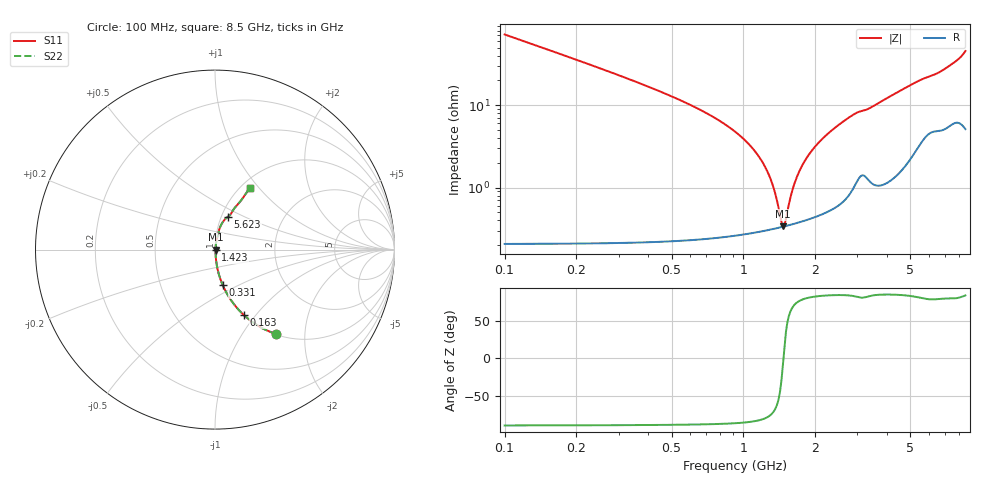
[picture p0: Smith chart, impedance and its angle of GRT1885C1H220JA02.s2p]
!Murata Part Number: GRT1885C1H220JA02
!These Parameters are Measured in Series Mode Connection
!Data Generated on Jun 19, 2026
!  o--ll--o
!Port1  Port2
!  o------o
!Operation Temp=25[degC], DC Bias Voltage=0[V]
!Freq. Start=100[MHz] Stop=9[GHz] 401[Steps]
# Hz S RI R 50
!Freq.(Hz) S11(Real) S11(Imag) S21(Real) S21(Imag) S12(Real) S12(Imag) S22(Real) S22(Imag)
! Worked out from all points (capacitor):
!   401 points, 100 MHz to 8.5 GHz, reference 50 ohm
!   read as one part in series: C = 22 pF near 142 MHz
!   lowest |Z| = 338 mohm at 1.465 GHz (marker M1)
!   series resonance near 1.471 GHz, so ESL is about 530 pH
!   S11 on the Smith chart (normalised r, x): 100 MHz: 1.00, -1.44; 163 MHz: 1.00, -0.88; 331 MHz: 1.00, -0.42; 1.423 GHz: 1.01, -0.01; 5.623 GHz: 1.07, +0.41; 8.5 GHz: 1.10, +0.90
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1e8  0.3419 -0.4729  0.6581 0.4729  0.6581 0.4729  0.3419 -0.4729
1.63e8  0.1624 -0.3664  0.8376 0.3664  0.8376 0.3664  0.1624 -0.3664
2.26e8  0.0906 -0.2837  0.9094 0.2837  0.9094 0.2837  0.0906 -0.2837
3.31e8  0.0432 -0.1982  0.9568 0.1982  0.9568 0.1982  0.0432 -0.1982
6.25e8  0.0112 -0.0937  0.9888 0.0937  0.9888 0.0937  0.0112 -0.0937
9.4e8  0.00469 -0.0453  0.9953 0.0453  0.9953 0.0453  0.00469 -0.0453
1.129e9  0.00355 -0.0263  0.9965 0.0263  0.9965 0.0263  0.00355 -0.0263
1.297e9  0.00324 -0.0124  0.9968 0.0124  0.9968 0.0124  0.00324 -0.0124
1.423e9  0.00329 -0.00326  0.9967 0.00326  0.9967 0.00326  0.00329 -0.00326
1.465e9  0.00335 -0.000392  0.9967 0.000392  0.9967 0.000392  0.00335 -0.000392
1.507e9  0.00342 0.0024  0.9966 -0.0024  0.9966 -0.0024  0.00342 0.0024
1.591e9  0.00362 0.00777  0.9964 -0.00777  0.9964 -0.00777  0.00362 0.00777
1.675e9  0.00388 0.0129  0.9961 -0.0129  0.9961 -0.0129  0.00388 0.0129
1.78e9  0.00428 0.019  0.9957 -0.019  0.9957 -0.019  0.00428 0.019
1.906e9  0.00486 0.026  0.9951 -0.026  0.9951 -0.026  0.00486 0.026
2.305e9  0.00743 0.0467  0.9926 -0.0467  0.9926 -0.0467  0.00743 0.0467
2.914e9  0.016 0.0754  0.984 -0.0754  0.984 -0.0754  0.016 0.0754
4.3e9  0.0308 0.1308  0.9692 -0.1308  0.9692 -0.1308  0.0308 0.1308
5.623e9  0.0715 0.1827  0.9285 -0.1827  0.9285 -0.1827  0.0715 0.1827
5.707e9  0.0745 0.1848  0.9255 -0.1848  0.9255 -0.1848  0.0745 0.1848
7.114e9  0.1137 0.2372  0.8863 -0.2372  0.8863 -0.2372  0.1137 0.2372
8.5e9  0.1964 0.3445  0.8036 -0.3445  0.8036 -0.3445  0.1964 0.3445
